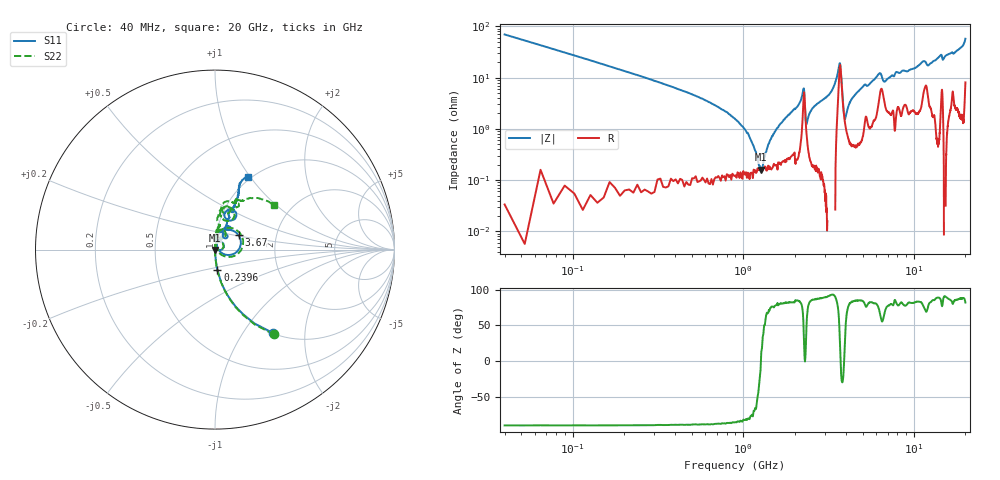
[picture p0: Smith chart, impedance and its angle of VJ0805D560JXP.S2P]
! VJ0805D560JXP
! DATE 10/29/2021  12:51
! CAPACITORS MOUNTED IN SERIES ON 25 MIL THICK MICROSTRIP SUBSTRATE
# GHz  S  MA  R  50.00
!  FREQ  S11M  S11A  S21M  S21A  S12M  S12A  S22M  S22A
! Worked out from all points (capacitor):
!   1601 points, 40 MHz to 20 GHz, reference 50 ohm
!   read as one part in series: C = 57.1 pF near 139.8 MHz
!   lowest |Z| = 159 mohm at 1.263 GHz (marker M1)
!   series resonance near 1.269 GHz, so ESL is about 280 pH
!   S11 on the Smith chart (normalised r, x): 40 MHz: 1.01, -1.38; 239.6 MHz: 1.00, -0.23; 3.67 GHz: 1.29, +0.21; 20 GHz: 0.97, +0.98
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0.04  0.5677 -55.1  0.8231 34.8  0.8201 34.8  0.5758 -55.2
0.2396  0.1117 -83.1  0.9926 6.3  0.9924 6.3  0.1128 -83.7
1.01305  0.01146 -82.3  0.9985 0.5  0.9983 0.4  0.01188 -85.2
1.26255  0.00277 -52.0  0.998 -0.1  0.9985 -0.1  0.002123 -62.0
1.36235  0.002382 28.3  0.9988 -0.3  0.9981 -0.3  0.001584 54.5
1.624325  0.009401 70.7  0.9977 -0.8  0.9974 -0.8  0.009747 83.2
2.1857  0.03554 76.6  0.9925 -2.3  0.9928 -2.4  0.03485 78.3
2.41025  0.01487 71.3  0.9962 -1.1  0.9957 -1.2  0.01416 82.7
3.370825  0.05277 83.5  1.001 -3.9  1.002 -4.0  0.06526 93.7
3.670225  0.1543 31.0  0.86 -5.7  0.8604 -5.8  0.1678 26.5
3.8823  0.02437 -15.0  0.9792 -0.0  0.9788 -0.0  0.01493 -27.2
3.969625  0.01743 25.4  0.9881 -0.8  0.9877 -0.9  0.01003 57.4
4.293975  0.03143 70.6  0.9935 -2.3  0.9937 -2.4  0.0349 90.0
5.0799  0.06356 65.5  0.9889 -4.2  0.9889 -4.3  0.06726 89.6
6.2775  0.1052 54.4  0.9544 -6.5  0.9547 -6.7  0.1183 69.7
6.70165  0.08143 53.0  0.9647 -4.5  0.9643 -4.6  0.06998 67.1
10.02  0.137 64.0  0.9688 -8.8  0.9672 -8.9  0.1407 80.9
11.34235  0.1339 54.0  0.9359 -11.3  0.9362 -11.5  0.2494 72.8
13.35083  0.2005 66.8  0.9669 -12.9  0.9668 -13.1  0.1969 82.0
16.68165  0.2478 66.4  0.9246 -18.0  0.925 -18.2  0.2868 64.1
19.22655  0.3683 69.0  0.9088 -24.6  0.9089 -24.9  0.311 61.2
20  0.4479 65.4  0.8092 -31.9  0.8081 -32.1  0.4124 36.8
